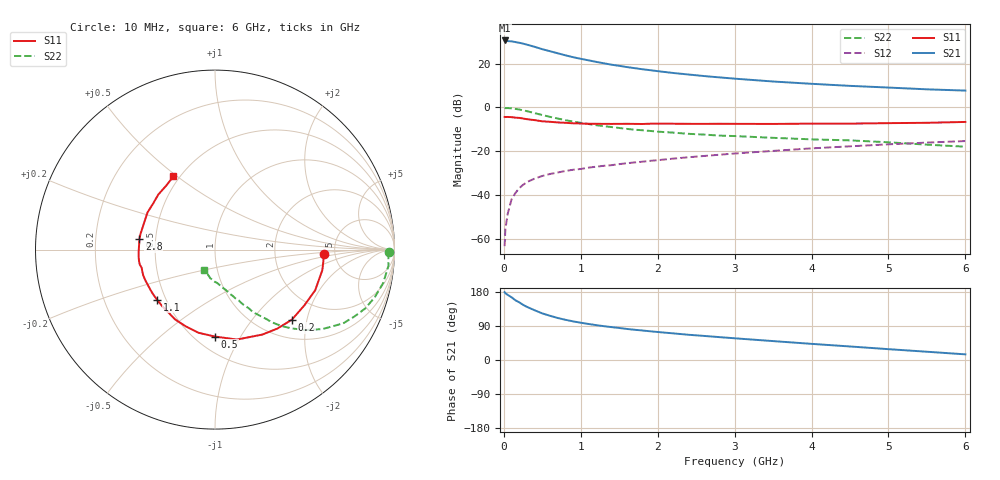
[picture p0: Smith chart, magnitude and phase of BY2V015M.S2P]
! SIEMENS Small Signal Semiconductors
! BFY420
! Si NPN RF SIEGET Grounded Emitter Transistor in MICRO-X
! VCE = 2 V  IC = 15 mA
! Common Emitter S-Parameters:  October  1996
# GHz  S  MA  R  50
!  f  S11  S21  S12  S22
! GHz  MAG  ANG  MAG  ANG  MAG  ANG  MAG  ANG
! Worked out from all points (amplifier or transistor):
!   36 points, 10 MHz to 6 GHz, reference 50 ohm
!   highest |S21| = 30.5 dB at 10 MHz (marker M1)
!   |S21| within 3 dB of that: start of sweep to 409.9 MHz
!   unconditionally stable (mu >= 1): 2.175 GHz to end of sweep
!   at 250 MHz: K = 0.25, MSG = 32.1 dB, |S12| = -35.2 dB
!   at 1.4 GHz: K = 0.86, MSG = 22.9 dB, |S12| = -26.2 dB
!   at 6 GHz: K = 1.08, MAG = 9.7 dB, |S12| = -15.3 dB
!   S11 on the Smith chart (normalised r, x): 10 MHz: 4.10, -0.35; 200 MHz: 1.38, -1.63; 500 MHz: 0.62, -0.78; 1.1 GHz: 0.45, -0.31; 2.8 GHz: 0.40, +0.06; 6 GHz: 0.46, +0.48
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0.01  0.61 -2.5  33.47 178.9  0.0007 87.8  0.9688 -0.8
0.02  0.6073 -4.8  33.41 176.1  0.0017 79.8  0.9662 -1.8
0.05  0.6089 -10.8  32.39 171.9  0.0038 86.8  0.9705 -5.3
0.1  0.6024 -22.1  31.89 165.5  0.0081 83.9  0.956 -11.1
0.15  0.5868 -32.0  30.76 157.7  0.0113 75.8  0.9294 -16.5
0.2  0.5795 -42.4  29.69 152.2  0.0146 73.6  0.8997 -21.3
0.25  0.5607 -51.7  28.3 145.6  0.0174 68.2  0.8601 -25.8
0.3  0.5418 -60.9  26.89 140.2  0.0201 66.0  0.8241 -29.9
0.4  0.5159 -76.3  23.99 131.3  0.0241 61.7  0.7434 -36.6
0.5  0.4843 -90.1  21.16 122.9  0.0277 58.8  0.6733 -41.7
0.7  0.4572 -111.1  17.11 110.9  0.0332 55.2  0.561 -49.2
0.8  0.4481 -119.8  15.38 106.1  0.0359 53.3  0.5149 -51.9
0.9  0.4367 -126.0  13.94 102.0  0.0383 53.5  0.4774 -53.7
1.1  0.4269 -139.2  11.82 95.1  0.0427 53.2  0.4202 -57.7
1.3  0.4238 -147.9  10.12 89.3  0.0471 52.8  0.3752 -60.2
1.6  0.425 -159.9  8.294 81.9  0.054 53.0  0.3257 -64.1
2.2  0.4272 -175.8  6.097 70.3  0.0686 52.1  0.2679 -70.2
2.8  0.4254 172.0  4.839 60.4  0.0841 49.6  0.2294 -75.6
3.5  0.4223 159.1  3.898 49.9  0.1029 45.8  0.204 -81.5
4.5  0.4295 143.6  3.102 35.7  0.1308 38.3  0.1785 -90.7
5.5  0.4482 127.3  2.588 21.8  0.159 29.4  0.1427 -106.9
6  0.4689 119.7  2.422 14.9  0.1723 24.7  0.1282 -118.8
